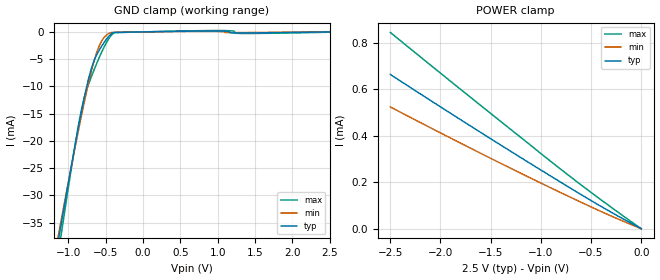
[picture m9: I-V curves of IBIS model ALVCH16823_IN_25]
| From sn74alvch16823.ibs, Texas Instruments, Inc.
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[Model]   ALVCH16823_IN_25
Model_type  Input
Vinl=0.7
Vinh=1.7
| variable   typ   min   max
C_comp   2.65pF   1.91pF   3.17pF
[Temperature Range]   40   100   -40
| Ambient temperature   25   85   -40
[Voltage range]   2.5   2.3   2.7
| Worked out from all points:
|   GND clamp passes 1 mA (typ) near -0.47 V on its own axis
[GND Clamp]
| ALVCH16823_IN_25
|   Voltage   I(typ)   I(min)   I(max)
-2.5V     -153.2mA   -143.6mA   -168.7mA
-1.15V    -39.47mA   -38.43mA   -41.94mA
-1.115V   -36.66mA   -35.85mA   -38.77mA
-1.085V   -34.27mA   -33.64mA   -36.06mA
-940mV    -22.97mA   -23.19mA   -23.22mA
-840mV    -15.61mA   -16.31mA   -15.24mA
-730mV    -8.578mA   -9.318mA   -9.607mA
-665mV    -5.593mA   -5.765mA   -7.269mA
-590mV    -3.421mA   -2.659mA   -4.792mA
-460mV    -821.1uA   -306.8uA   -1.275mA
-375mV    -100.8uA   -82.47uA   -137.6uA
2.5V      35.46pA    35.81uA    -58.91uA
[POWER Clamp]
| ALVCH16823_IN_25
|   Voltage   I(typ)   I(min)   I(max)
-2.5V     663.5uA    523.6uA    844.3uA
-1.58V    408.7uA    320uA      523.4uA
-820mV    204.6uA    158.8uA    261.8uA
-400mV    95.75uA    73.84uA    124uA
-31.15fV  35.46pA    139.5pA    38.15pA
